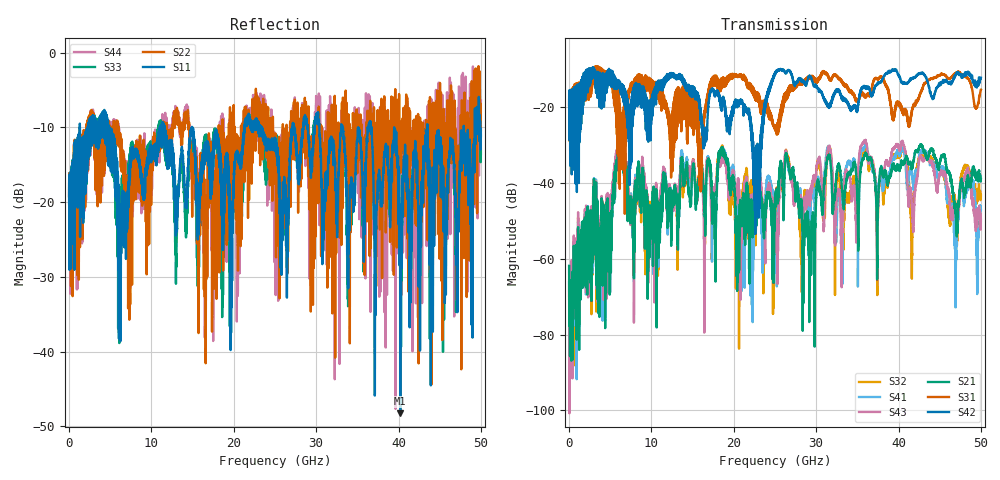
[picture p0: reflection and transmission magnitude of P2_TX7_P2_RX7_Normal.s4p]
!Keysight Technologies,N5225B,MY57041031,A.13.20.10
!Date: Friday, May 31, 2019 11:38:09
!Correction: S11(Full 4 Port(1,2,3,4))
!S12(Full 4 Port(1,2,3,4))
!S13(Full 4 Port(1,2,3,4))
!S14(Full 4 Port(1,2,3,4))
!S21(Full 4 Port(1,2,3,4))
!S22(Full 4 Port(1,2,3,4))
!S23(Full 4 Port(1,2,3,4))
!S24(Full 4 Port(1,2,3,4))
!S31(Full 4 Port(1,2,3,4))
!S32(Full 4 Port(1,2,3,4))
!S33(Full 4 Port(1,2,3,4))
!S34(Full 4 Port(1,2,3,4))
!S41(Full 4 Port(1,2,3,4))
!S42(Full 4 Port(1,2,3,4))
!S43(Full 4 Port(1,2,3,4))
!S44(Full 4 Port(1,2,3,4))
!S4P File: Measurements: <S11,S12,S13,S14>,
!<S21,S22,S23,S24>,
!<S31,S32,S33,S34>,
!<S41,S42,S43,S44>:
# Hz S  dB  R 50.0
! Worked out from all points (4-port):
!   5000 points, 10 MHz to 50 GHz, reference 50 ohm
!   strongest paths, dB at 10 MHz, 12.51 GHz, 25.01 GHz, 37.51 GHz, 50 GHz:
!     S42: -19.4, -12.1, -11.4, -13.7, -12.3
!     S31: -19.6, -22.5, -25.6, -12.7, -15.4
!     S21: -61.9, -45.8, -43.9, -46.2, -39.0
!     S43: -69.7, -45.2, -48.2, -46.4, -49.7
!     S41: -66.2, -45.9, -48.1, -42.7, -47.0
!     S32: -70.6, -45.4, -44.8, -47.7, -43.4
!   lowest |S11| = -48.3 dB at 40.21 GHz (marker M1), VSWR 1.01, Z = 49.7 + j0.232 ohm
!   |S11| at or under -10 dB: 4.911 GHz to 11.03 GHz (6.119 GHz wide, 76.8 % of centre); 14.96 GHz to 21.26 GHz (6.296 GHz wide, 34.8 % of centre); 43.5 GHz to 47.92 GHz (4.413 GHz wide, 9.65 % of centre)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
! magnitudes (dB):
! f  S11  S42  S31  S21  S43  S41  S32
! 10 MHz  -20.2  -19.4  -19.6  -61.9  -69.7  -66.2  -70.6
! 6.14 GHz  -28.6  -13.7  -20.3  -29.4  -28.7  -29.0  -29.1
! 9.79 GHz  -13.1  -18.3  -15.7  -49.3  -48.6  -53.6  -46.5
! 18.76 GHz  -17.9  -18.1  -13.6  -31.5  -32.3  -31.3  -31.2
! 22.15 GHz  -9.3  -24.8  -15.2  -48.0  -45.0  -58.5  -41.4
! 40.21 GHz  -48.3  -12.4  -19.8  -36.2  -31.0  -32.4  -32.7
! 50 GHz  -11.2  -12.3  -15.4  -39.0  -49.7  -47.0  -43.4
